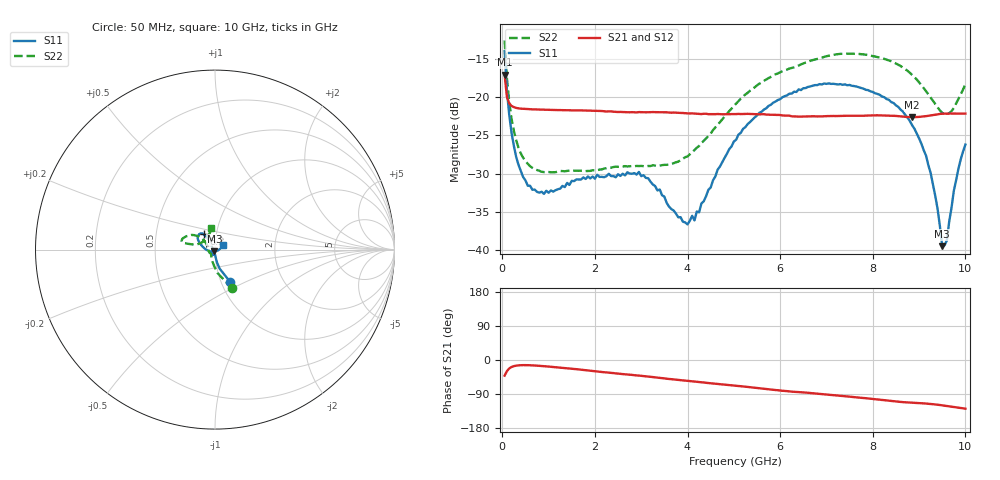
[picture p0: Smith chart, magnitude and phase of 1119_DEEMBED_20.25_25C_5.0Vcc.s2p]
!Hittite Microwave Corp.
!Digital Attenuator/PhaseShifter Rev 1.4.0
!Filename: C:\DATA\DATA\1119_DEEMBED_20.25_25C_5.0Vcc.s2p
!VNA ID: Agilent Technologies,N5224A,MY51441122,A.10.45.03
!Device type:
!2 Port Calibration.
!Temp(C): 25
!Lot Number:
!Serial Number:
!Operator:
!Misc:
!Attenuator:  20.250
# GHZ S DB R 50.0
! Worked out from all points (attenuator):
!   200 points, 50 MHz to 10 GHz, reference 50 ohm
!   highest |S21| = -17.06 dB at 50 MHz (marker M1); lowest = -22.6 dB at 8.85 GHz (marker M2)
!   lowest |S11| = -39.5 dB at 9.5 GHz (marker M3), VSWR 1.02, Z = 49.7 - j1.01 ohm
!   |S11| at or under -10 dB: start of sweep to end of sweep
!   |S22| runs from -29.8 to -12.6 dB; largest |S21 - S12| = 0.00028
!   S11 on the Smith chart (normalised r, x): 50 MHz: 1.10, -0.42; 6.2 GHz: 0.87, +0.15; 10 GHz: 1.09, +0.05
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0.05  -13.98 -64.7  -17.06 -41.2  -17.06 -41.3  -12.59 -66.4
0.1  -19.16 -76.1  -19.99 -29.3  -19.99 -29.3  -17.55 -83.3
0.2  -24.67 -83.0  -21.15 -18.4  -21.15 -18.4  -22.83 -100.0
0.35  -28.86 -86.2  -21.47 -14.1  -21.47 -14.1  -26.62 -114.0
0.55  -31.59 -90.2  -21.57 -13.7  -21.57 -13.7  -28.72 -125.5
0.9  -32.66 -96.2  -21.64 -16.3  -21.64 -16.3  -29.81 -134.7
1.75  -30.51 -111.8  -21.75 -26.3  -21.75 -26.3  -29.64 -139.5
2.95  -29.79 -116.5  -21.96 -41.1  -21.98 -41.1  -29.02 -158.4
3.4  -32.08 -130.9  -21.98 -47.1  -21.99 -47.1  -28.96 -171.8
3.9  -36.30 -171.5  -22.08 -54.0  -22.09 -54.1  -28.07 168.5
4.15  -36.13 159.1  -22.15 -57.2  -22.16 -57.3  -26.94 157.7
5.05  -25.57 120.9  -22.22 -67.8  -22.23 -67.8  -20.84 139.7
6.2  -19.55 125.5  -22.43 -83.0  -22.45 -83.0  -16.26 147.9
6.7  -18.52 131.9  -22.51 -87.7  -22.52 -87.7  -15.16 154.6
8.35  -20.36 155.6  -22.43 -107.4  -22.43 -107.4  -15.21 168.0
8.85  -23.68 168.8  -22.64 -112.7  -22.63 -112.7  -17.10 167.6
9.25  -29.94 -163.8  -22.40 -116.0  -22.41 -116.0  -20.07 161.9
9.400001  -34.65 -141.2  -22.26 -118.0  -22.27 -118.0  -21.35 153.4
9.5  -39.50 -105.9  -22.18 -119.8  -22.20 -119.8  -22.06 144.0
9.6  -38.74 -44.0  -22.17 -121.5  -22.18 -121.5  -22.21 132.9
9.75  -32.26 3.4  -22.14 -124.0  -22.16 -124.0  -21.41 115.5
10  -26.21 29.2  -22.16 -128.4  -22.17 -128.4  -18.33 99.5
